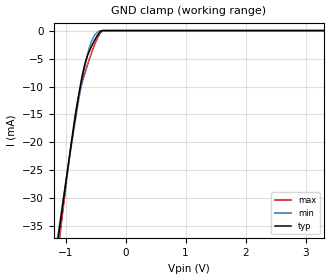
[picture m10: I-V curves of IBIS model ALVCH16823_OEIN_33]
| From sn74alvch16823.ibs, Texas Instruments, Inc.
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[Model]   ALVCH16823_OEIN_33
Model_type  Input
Vinl=0.8
Vinh=2.145
| variable   typ   min   max
C_comp   2.49pF   1.82pF   3.18pF
[Temperature Range]   40   100   -40
| Ambient temperature   25   85   -40
[Voltage range]   3.3   3   3.6
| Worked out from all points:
|   GND clamp passes 1 mA (typ) near -0.48 V on its own axis
[GND Clamp]
| ALVCH16823_OEIN_33
|   Voltage   I(typ)   I(min)   I(max)
-3.3V     -222.4mA   -207.7mA   -245.4mA
-1.125V   -37.37mA   -36.52mA   -39.57mA
-1.095V   -34.97mA   -34.31mA   -36.86mA
-1.065V   -32.59mA   -32.11mA   -34.16mA
-855mV    -16.59mA   -17.25mA   -16.23mA
-790mV    -12.12mA   -12.96mA   -12.11mA
-720mV    -7.968mA   -8.671mA   -9.142mA
-660mV    -5.336mA   -5.456mA   -7.005mA
-585mV    -3.229mA   -2.435mA   -4.541mA
-440mV    -448uA     -97.75uA   -766.1uA
-375mV    -85.17nA   -8.524uA   -4.38uA
3.3V      45.43pA    164.4pA    42.9pA
